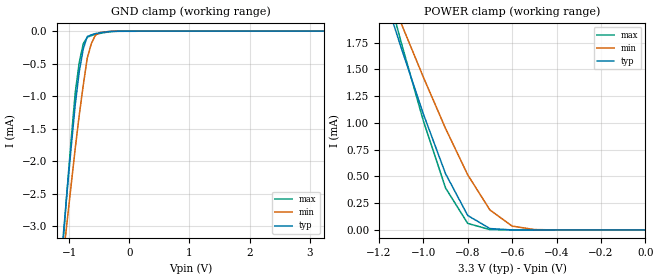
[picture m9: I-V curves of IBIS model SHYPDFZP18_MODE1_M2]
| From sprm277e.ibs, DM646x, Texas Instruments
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|   Model Cell SHYPDFZP18_MODE1_M2
[Model]   SHYPDFZP18_MODE1_M2
Model_type   Input
Polarity   Non-Inverting
Vinl =  0.8V
Vinh =  2V
C_comp   0.7732787p   0.7118968p   0.8502484p
[Model Spec]
Vinl   0.8V   0.8V   0.8V
Vinh   2V   2V   2V
[Temperature Range]   25   105   0
[Voltage Range]   3.3   3.14   3.47
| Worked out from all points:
|   GND clamp passes 1 mA (typ) near -0.88 V on its own axis
|   POWER clamp passes 1 mA (typ) near -0.98 V on its own axis
[POWER_clamp]
|   voltage   I(typ)   I(min)   I(max)
-3.3V     16.09mA    13.57mA    18.63mA
-1.133V   1.92mA     2.103mA    2.013mA
-1.1V     1.705mA    1.931mA    1.755mA
-1.067V   1.498mA    1.764mA    1.511mA
-1V       1.085mA    1.428mA    1.021mA
-900mV    526.2uA    948.7uA    393.3uA
-800mV    135.4uA    515.1uA    61.39uA
-700mV    13.19uA    186.7uA    3.59uA
-600mV    617.7nA    36.18uA    585.6nA
-500mV    119.5nA    3.806uA    513.7nA
0V        95.63nA    68.71nA    458.7nA
[GND_clamp]
|   voltage   I(typ)   I(min)   I(max)
-3.3V     -27.74mA   -23.32mA   -31.25mA
-1.1V     -3.146mA   -3.479mA   -3.223mA
-1.033V   -2.444mA   -2.909mA   -2.417mA
-966.7mV  -1.771mA   -2.349mA   -1.659mA
-900mV    -1.127mA   -1.801mA   -946.7uA
-833.3mV  -621.6uA   -1.293mA   -479.4uA
-766.7mV  -273.8uA   -830.3uA   -194.9uA
-700mV    -83.63uA   -413.1uA   -93.23uA
-633.3mV  -57.76uA   -195.2uA   -70.2uA
-566.7mV  -39.01uA   -65.53uA   -51.58uA
-433.3mV  -18.12uA   -15.12uA   -25.7uA
3.233V    94.38nA    69.82nA    436.5nA
